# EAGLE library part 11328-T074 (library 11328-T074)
Power Transformers Flyback Transformer for LT8316 Source: Datasheet
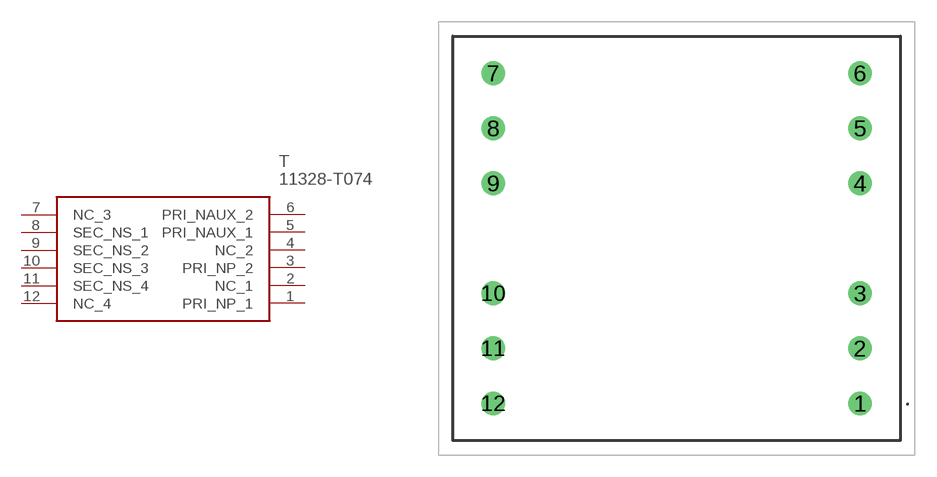
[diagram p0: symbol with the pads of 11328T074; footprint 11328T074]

Designator prefix T

## 11328-T074 (Description: Power Transformers Flyback Transformer for LT8316; Height: 23.5mm; Manufacturer_Name: Sumida; Manufacturer_Part_Number: 11328-T074; Mouser_Part_Number: 851-11328-T074; Mouser_Price-Stock: https://www.mouser.co.uk/ProductDetail/Sumida/11328-T074?qs=DRkmTr78QASTM1HSK8DGZg%3D%3D)  [11328T074]
1  PRI_NP_1
2  NC_1
3  PRI_NP_2
4  NC_2
5  PRI_NAUX_1
6  PRI_NAUX_2
7  NC_3
8  SEC_NS_1
9  SEC_NS_2
10  SEC_NS_3
11  SEC_NS_4
12  NC_4

## Footprint 11328T074 (pad centres in mm)
11328-T074-1
drill 1.1 pad 1.65: 1 0,0; 2 0,3.81; 3 0,7.62; 4 0,15.24; 5 0,19.05; 6 0,22.86; 7 -25.4,22.86; 8 -25.4,19.05; 9 -25.4,15.24; 10 -25.4,7.62; 11 -25.4,3.81; 12 -25.4,0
